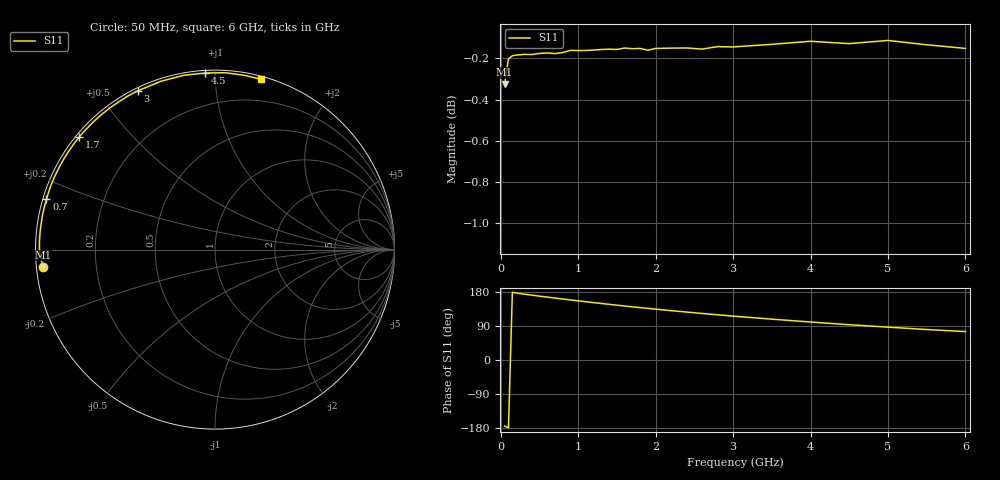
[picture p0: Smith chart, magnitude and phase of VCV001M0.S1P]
! Infineon Technologies  Discrete & RF Semiconductors
! BBY 56-03
! Si Tuning Diode in SOD323
! VR =
! S-Parameters:  June  1999
# GHz  S  MA  R  50
!  f  S11
! GHz  MAG  ANG
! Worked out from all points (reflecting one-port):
!   34 points, 50 MHz to 6 GHz, reference 50 ohm
!   lowest |S11| = -0.3 dB at 50 MHz (marker M1), VSWR 53.47, Z = 0.938 - j2.53 ohm
!   phase of S11 starts at -174 deg and turns -111 deg over the sweep
!   S11 on the Smith chart (normalised r, x): 50 MHz: 0.02, -0.05; 700 MHz: 0.01, +0.15; 1.7 GHz: 0.01, +0.36; 3 GHz: 0.01, +0.63; 4.5 GHz: 0.01, +0.95; 6 GHz: 0.02, +1.30
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0.05  0.9633 -174.2
0.1  0.977 -178.9
0.15  0.9787 178.7
0.2  0.979 176.8
0.3  0.9795 173.8
0.4  0.9794 171.1
0.5  0.98 168.5
0.7  0.9799 163.4
0.8  0.9805 160.9
0.9  0.9817 158.5
1  0.9816 156.1
1.2  0.9818 151.4
1.4  0.9823 146.9
1.6  0.9829 142.5
1.7  0.9826 140.3
1.8  0.9827 138.2
2  0.9827 134.2
2.2  0.9829 130.2
2.4  0.983 126.5
2.6  0.9824 122.8
2.8  0.9837 119.3
3  0.9835 115.8
3.5  0.985 107.8
4  0.9867 100.2
4.5  0.9854 93.1
5  0.9871 86.7
5.5  0.9847 80.4
6  0.9827 75.0
